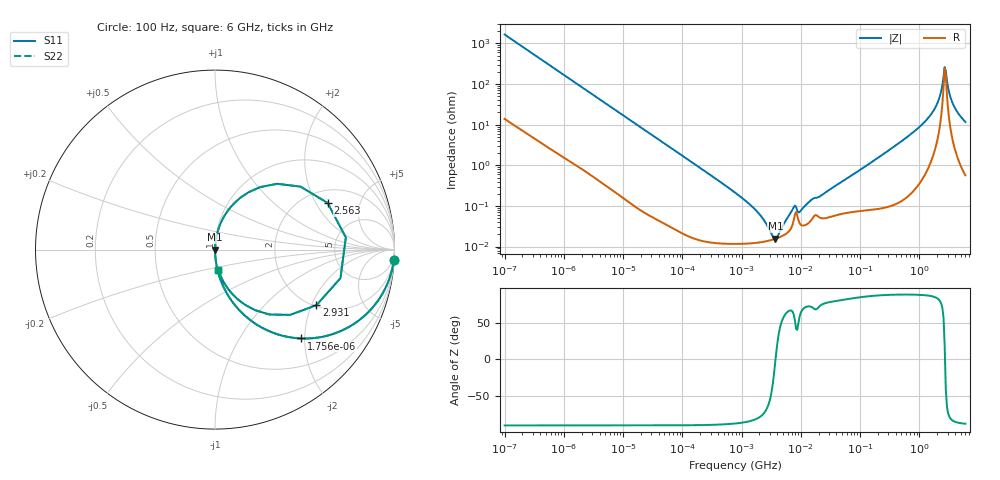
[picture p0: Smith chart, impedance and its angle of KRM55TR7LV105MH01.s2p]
!Murata Part Number: KRM55TR7LV105MH01
!These Parameters are Measured in Series Mode Connection
!Data Generated on Jan 08, 2026
!  o--ll--o
!Port1  Port2
!  o------o
!Operation Temp=25[degC], DC Bias Voltage=0[V]
!Freq. Start=100[Hz] Stop=6[GHz] 401[Steps]
# Hz S RI R 50
!Freq.(Hz) S11(Real) S11(Imag) S21(Real) S21(Imag) S12(Real) S12(Imag) S22(Real) S22(Imag)
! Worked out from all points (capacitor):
!   401 points, 100 Hz to 6 GHz, reference 50 ohm
!   read as one part in series: C = 956 nF near 109 Hz
!   lowest |Z| = 15.6 mohm at 3.712 MHz (marker M1)
!   series resonance near 3.74 MHz, so ESL is about 1.9 nH
!   S11 on the Smith chart (normalised r, x): 100 Hz: 1, -33; 1.756 kHz: 1.02, -1.92; 2.563 GHz: 2.61, +2.52; 2.931 GHz: 2.05, -2.17; 6 GHz: 1.01, -0.23
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100  0.9959 -0.0599  0.00411 0.0599  0.00411 0.0599  0.9959 -0.0599
548  0.9013 -0.2939  0.0987 0.2939  0.0987 0.2939  0.9013 -0.2939
1756  0.4805 -0.4948  0.5195 0.4948  0.5195 0.4948  0.4805 -0.4948
2008  0.4152 -0.488  0.5848 0.488  0.5848 0.488  0.4152 -0.488
6151  0.0731 -0.2557  0.9269 0.2557  0.9269 0.2557  0.0731 -0.2557
40335  0.00224 -0.0425  0.9978 0.0425  0.9978 0.0425  0.00224 -0.0425
774597  0.000121 -0.00214  0.9999 0.00214  0.9999 0.00214  0.000121 -0.00214
1896632  0.000125 -0.000675  0.9999 0.000675  0.9999 0.000675  0.000125 -0.000675
3712478  0.000156 -6.6e-06  0.9998 6.6e-06  0.9998 6.6e-06  0.000156 -6.6e-06
7599586  0.000449 0.000813  0.9996 -0.000813  0.9996 -0.000813  0.000449 0.000813
9941735  0.000347 0.00068  0.9997 -0.00068  0.9997 -0.00068  0.000347 0.00068
1.555665e7  0.000484 0.00138  0.9995 -0.00138  0.9995 -0.00138  0.000484 0.00138
3.124326e8  0.00154 0.0239  0.9985 -0.0239  0.9985 -0.0239  0.00154 0.0239
9.569533e8  0.00991 0.0814  0.9901 -0.0814  0.9901 -0.0814  0.00991 0.0814
1.712697e9  0.0585 0.1977  0.9415 -0.1977  0.9415 -0.1977  0.0585 0.1977
2.240541e9  0.2522 0.3485  0.7478 -0.3485  0.7478 -0.3485  0.2522 0.3485
2.562649e9  0.6275 0.2599  0.3725 -0.2599  0.3725 -0.2599  0.6275 0.2599
2.679998e9  0.7289 0.0679  0.2711 -0.0679  0.2711 -0.0679  0.7289 0.0679
2.931063e9  0.5649 -0.31  0.4351 0.31  0.4351 0.31  0.5649 -0.31
3.205649e9  0.3028 -0.3614  0.6972 0.3614  0.6972 0.3614  0.3028 -0.3614
3.666503e9  0.1278 -0.2778  0.8722 0.2778  0.8722 0.2778  0.1278 -0.2778
6e9  0.0188 -0.1137  0.9812 0.1137  0.9812 0.1137  0.0188 -0.1137
